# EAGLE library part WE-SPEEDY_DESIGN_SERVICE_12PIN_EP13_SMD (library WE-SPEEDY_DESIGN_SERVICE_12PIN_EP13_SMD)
WE-Speedy Design Service, 12 Pin - Any application that fits package style - Switch Mode Power: Flyback, Forward, Push-Pull, Coupled Inductor -- Telecom Applications: xDSL, POTS Splitter Inductors
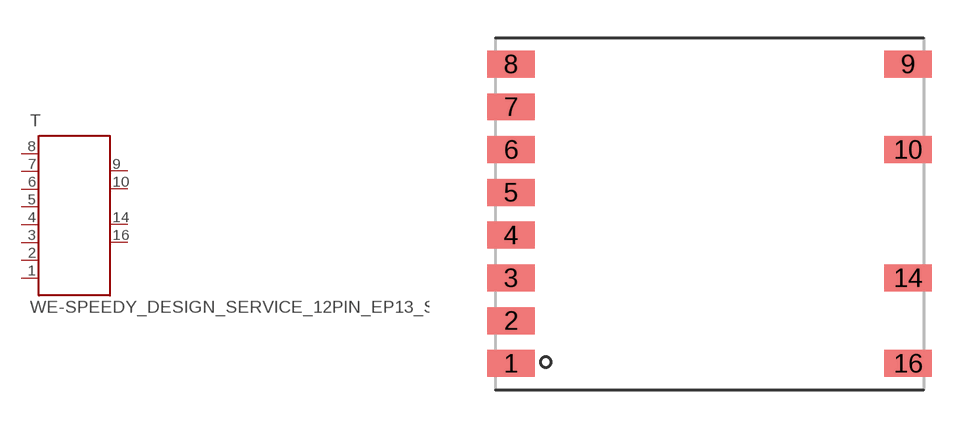
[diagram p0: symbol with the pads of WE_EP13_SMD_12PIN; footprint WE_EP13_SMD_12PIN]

Designator prefix T

## WE-SPEEDY_DESIGN_SERVICE_12PIN_EP13_SMD-750311856 (MPN: 750311856; OC_FARNELL: 1895748; OC_NEWARK: 47T5866; PACKAGE: EP13_SMD; SUPPLIER: Würth Elektronik eiSos GmbH)  [WE_EP13_SMD_12PIN]
1  1  pas
2  2  pas
3  3  pas
4  4  pas
5  5  pas
6  6  pas
7  7  pas
8  8  pas
9  9  pas
10  10  pas
14  11  pas
16  12  pas

## Footprint WE_EP13_SMD_12PIN (pad centres in mm)
Transformer, EP13 SMD 12 Pin
smd 1.88 x 1.07: 1 -7.885,-5.95; 2 -7.885,-4.25; 3 -7.885,-2.55; 4 -7.885,-0.85; 5 -7.885,0.85; 6 -7.885,2.55; 7 -7.885,4.25; 8 -7.885,5.95; 9 7.885,5.95; 10 7.885,2.55; 14 7.885,-2.55; 16 7.885,-5.95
